PROGRAM RobotBasic
VAR
	// 使能、复位所有轴
	benable						: BOOL;                            //使能信号
	bReset                      : BOOL;                            //复位信号
	fbpower						: ARRAY [1..7] OF Tc2_MC2.MC_Power;//使能功能块
	fbReset					    : ARRAY [1..7] OF Tc2_MC2.MC_Reset;//复位功能块
	IsAllAxisReady              : BOOL;                            //使能标志位
	
    // 机器人轴组
	stAxesConfig				: ST_KinAxes;                    
	
    // 机器人变量
	in_stKinToPlc	AT %I*		: NcToPlc_NciChannel_Ref;
	out_stPlcToKin	AT %Q*		: PLCTONC_NCICHANNEL_REF;
	
	// 耦合复位机器人功能块
	fbConfigKinGroup			: FB_KinConfigGroup;  
	fbResetKinGroup             : FB_KinResetGroup;
	
    // 机器人相关标志为
	xUserConfigGroup			: BOOL := FALSE;                   //耦和触发位
	xUserResetGroup			    : BOOL := FALSE;                   //复位触发位
	xUserCartesianMode			: BOOL := TRUE;  
	IsxUserKinGroupReady        : BOOL;                            //机器人轴组是否耦合
		
    // 其它
	i							: INT;//循环用变量
	AxisError                   : BOOL;//报错判断
	fbSetCposition              : MC_SetPosition;
END_VAR

EnableRobot();//调用机器人使能Action
ResetRobot();//调用机器人复位Action

ACTION EnableRobot:
//调用耦合机器人轴组功能块
fbConfigKinGroup(
	bExecute					:= xUserConfigGroup, 
	bCartesianMode			    := xUserCartesianMode, 
	stAxesList					:= stAxesConfig, 
	stKinRefIn					:= in_stKinToPlc
);

fbSetCposition(
	Axis:=AxisArray[4] ,  
	Position:=0 , 
);

//轮询读取轴的状态
FOR i := 1 TO 7 BY 1 DO
    AxisArray[i].ReadStatus();
END_FOR

// 使能所有轴
IF benable THEN
	FOR i := 1 TO 7 BY 1 DO//用For语句轮询进行使能
		fbpower[i](
			Axis:= AxisArray[i], 
			Enable:= TRUE, 
			Enable_Positive:= TRUE, 
			Enable_Negative:= TRUE, 
			Override:= 100);
	END_FOR
	
// 以互锁的方式判断是能是否成功，是否有报错
	IF fbpower[1].Status AND fbpower[2].Status AND fbpower[3].Status AND fbpower[4].Status AND fbpower[5].Status AND fbpower[6].Status AND fbpower[7].Status THEN
	   IF NOT AxisArray[1].Status.Error AND NOT AxisArray[2].Status.Error AND NOT AxisArray[3].Status.Error AND NOT AxisArray[4].Status.Error AND NOT AxisArray[5].Status.Error
		  AND NOT AxisArray[6].Status.Error AND NOT AxisArray[7].Status.Error THEN
		  AxisError:=FALSE;
          IsAllAxisReady:=TRUE;//若所有轴是能成功，则使能标志位置位
          benable := FALSE;
		  fbSetCposition.Execute:=TRUE;
	   ELSE
		  AxisError:=TRUE;//若有轴报错，则报错标志位置位
		  IsAllAxisReady:=FALSE;
		  benable := FALSE;
	   END_IF
	END_IF
END_IF
	 
// 将3个物理轴与笛卡尔坐标系轴注入机器人轴组
stAxesConfig.nAxisIdsAcs[1]		:= AxisArray[1].NcToPlc.AxisId;
stAxesConfig.nAxisIdsAcs[2]		:= AxisArray[2].NcToPlc.AxisId;
stAxesConfig.nAxisIdsAcs[3]		:= AxisArray[3].NcToPlc.AxisId;
stAxesConfig.nAxisIdsMcs[1]		:= AxisArray[5].NcToPlc.AxisId;
stAxesConfig.nAxisIdsMcs[2]		:= AxisArray[6].NcToPlc.AxisId;
stAxesConfig.nAxisIdsMcs[3]		:= AxisArray[7].NcToPlc.AxisId;

//使用功能块耦合轴组
IF xUserConfigGroup=TRUE THEN
   IF fbConfigKinGroup.bDone THEN
	  IsxUserKinGroupReady:=TRUE;//判断是否耦合成功，若成功则标志位置位
	  xUserConfigGroup:=FALSE;
   END_IF
END_IF

IF fbSetCposition.Done THEN
   fbSetCposition.Execute:=false;
END_IF
END_ACTION

ACTION ResetRobot:
//调用轴组复位功能块
fbResetKinGroup(
	bExecute                    :=xUserResetGroup, 
	nItpChannelId               :=5 , 
	stKinRefIn                  :=in_stKinToPlc , 
	stAxesList                  :=stAxesConfig , 
 );

//判断轴是否有报错
IF   AxisArray[1].Status.Error OR AxisArray[2].Status.Error OR AxisArray[3].Status.Error OR AxisArray[4].Status.Error 
	 OR AxisArray[5].Status.Error OR AxisArray[6].Status.Error OR  AxisArray[7].Status.Error THEN
     IsAllAxisReady:=FALSE;
     AxisError:=TRUE;
	 IsxUserKinGroupReady:=FALSE;
END_IF 

// 复位所有轴的指令
IF bReset THEN
	FOR i := 1 TO 7 BY 1 DO
		fbReset[i](
            Axis:= AxisArray[i], 
			Execute:= TRUE);
	END_FOR
//复位成功后使能并复位触发位
	IF fbReset[1].Done AND fbReset[2].Done  AND fbReset[3].Done  AND fbReset[4].Done  AND fbReset[5].Done  AND fbReset[6].Done  AND fbReset[7].Done THEN
	   bReset:= FALSE;
	   benable:= TRUE;
	   FOR i := 1 TO 7 BY 1 DO
	       fbReset[i](
            Axis:= AxisArray[i], 
			Execute:= FALSE);
	   END_FOR
	END_IF 
END_IF

//在轴报错后，同时也要用功能块对轴组进行复位
IF xUserResetGroup=TRUE THEN 
   IF fbResetKinGroup.bDone THEN
	  xUserConfigGroup:=TRUE;
	  xUserResetGroup:=FALSE;
	  IsxUserKinGroupReady:=TRUE;
   END_IF
END_IF
END_ACTION

END_PROGRAM
